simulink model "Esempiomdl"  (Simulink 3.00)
settings: Solver=ode45  StartTime=0.0  StopTime=50.0  RelTol=1e-3
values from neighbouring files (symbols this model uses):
  A = 0.01    [Esempio.m]
  b = 0.1    [Esempio.m]
  Cm = 0.001    [Esempio.m]
  Km = 10    [Esempio.m]    (also in Pompa.m = 0.00651965811966)
  Kv = 1    [Esempio.m]
  mp = 1    [Esempio.m]
  Pin = 10    [Esempio.m]
libraries: cstblocks x2

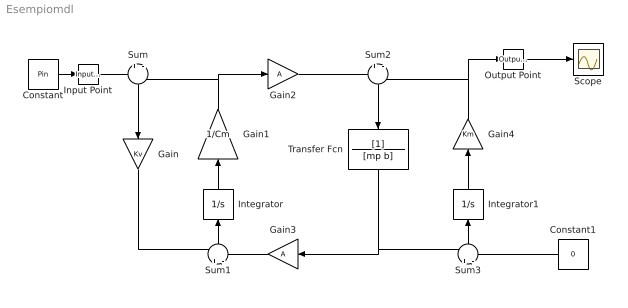
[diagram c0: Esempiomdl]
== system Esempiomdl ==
  Constant : Constant  Value=Pin
  Constant1 : Constant  Orientation=left  Value=0
  Gain : Gain  Orientation=down  Gain=Kv  SaturateOnIntegerOverflow=on
  Gain1 : Gain  Orientation=up  Gain=1/Cm  SaturateOnIntegerOverflow=on
  Gain2 : Gain  Gain=A  SaturateOnIntegerOverflow=on
  Gain3 : Gain  Orientation=left  Gain=A  SaturateOnIntegerOverflow=on
  Gain4 : Gain  Orientation=up  Gain=Km  SaturateOnIntegerOverflow=on
  Input Point : cstblocks/Input Point  PerturbationValue=0
  Integrator : Integrator  Orientation=up  ExternalReset=none  InitialConditionSource=internal  InitialCondition=0  LimitOutput=off  UpperSaturationLimit=inf  LowerSaturationLimit=-inf  ShowSaturationPort=off  ShowStatePort=off  AbsoluteTolerance=auto
  Integrator1 : Integrator  Orientation=up  ExternalReset=none  InitialConditionSource=internal  InitialCondition=0  LimitOutput=off  UpperSaturationLimit=inf  LowerSaturationLimit=-inf  ShowSaturationPort=off  ShowStatePort=off  AbsoluteTolerance=auto
  Output Point : cstblocks/Output Point  SigprobeOutputIndex=1
  Scope : Scope
  Sum : Sum  Orientation=down  Inputs=+|-  SaturateOnIntegerOverflow=on
  Sum1 : Sum  Orientation=up  Inputs=+|-  SaturateOnIntegerOverflow=on
  Sum2 : Sum  Orientation=down  Inputs=+|-  SaturateOnIntegerOverflow=on
  Sum3 : Sum  Orientation=up  Inputs=+|-  SaturateOnIntegerOverflow=on
  Transfer Fcn : TransferFcn  Orientation=down  Numerator=[1]  Denominator=[mp b]
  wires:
  Sum/1 -> Gain/1
  Gain/1 -> Sum1/1
  Sum1/1 -> Integrator/1
  Integrator/1 -> Gain1/1
  Gain1/1 -> Sum/2, Gain2/1
  Gain3/1 -> Sum1/2
  Gain2/1 -> Sum2/1
  Sum2/1 -> Transfer Fcn/1
  Integrator1/1 -> Gain4/1
  Sum3/1 -> Integrator1/1
  Transfer Fcn/1 -> Gain3/1, Sum3/1
  Constant1/1 -> Sum3/2
  Gain4/1 -> Sum2/2, Output Point/1
  Constant/1 -> Input Point/1
  Input Point/1 -> Sum/1
  Output Point/1 -> Scope/1
